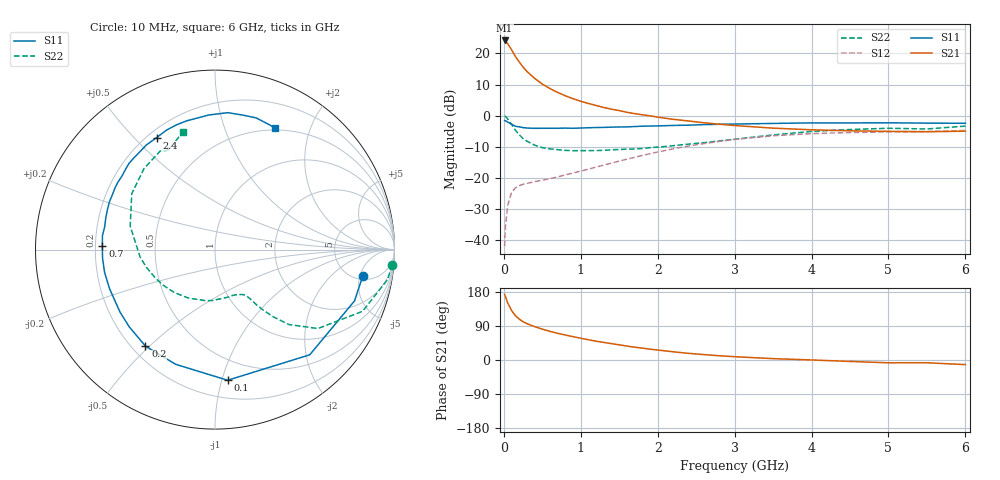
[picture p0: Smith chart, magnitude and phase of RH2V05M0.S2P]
! SIEMENS Small Signal Semiconductors
! BFR106
! Si NPN RF Bipolar Junction Transistor in SOT23
! VCE = 2 V  IC = 5 mA
! Common Emitter S-Parameters:  August  1996
# GHz  S  MA  R  50
!  f  S11  S21  S12  S22
! GHz  MAG  ANG  MAG  ANG  MAG  ANG  MAG  ANG
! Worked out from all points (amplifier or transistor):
!   36 points, 10 MHz to 6 GHz, reference 50 ohm
!   highest |S21| = 24.2 dB at 10 MHz (marker M1)
!   |S21| within 3 dB of that: start of sweep to 100.4 MHz
!   unconditionally stable (mu >= 1): 608.3 MHz to 2.204 GHz; 4.196 GHz to end of sweep
!   at 250 MHz: K = 0.51, MSG = 18.8 dB, |S12| = -22.1 dB
!   at 1.4 GHz: K = 1.17, MAG = 6.2 dB, |S12| = -15.2 dB
!   at 6 GHz: K = 1.03, MAG = -1.1 dB, |S12| = -4.7 dB
!   S11 on the Smith chart (normalised r, x): 10 MHz: 5.59, -5.56; 100 MHz: 0.33, -1.04; 200 MHz: 0.25, -0.49; 700 MHz: 0.23, +0.02; 2.4 GHz: 0.24, +0.58; 6 GHz: 0.48, +1.50
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0.01  0.8362 -10.3  16.19 173.1  0.008 87.6  0.9906 -4.9
0.02  0.8282 -20.2  15.84 167.8  0.016 80.0  0.9764 -9.8
0.05  0.7888 -48.0  14.34 150.7  0.0362 66.2  0.8911 -22.7
0.1  0.7313 -84.5  11.48 130.8  0.0583 51.0  0.7225 -37.5
0.15  0.6756 -109.0  8.952 116.8  0.0692 42.0  0.5864 -45.4
0.2  0.6627 -125.8  7.302 108.0  0.075 37.8  0.4952 -49.1
0.25  0.643 -138.0  6.043 100.9  0.0789 35.9  0.4281 -51.5
0.3  0.6336 -146.6  5.141 96.0  0.0817 35.5  0.3898 -52.9
0.4  0.6266 -159.7  3.982 88.1  0.0872 36.3  0.3362 -54.5
0.5  0.6282 -168.4  3.223 81.4  0.0918 38.5  0.3065 -56.2
0.6  0.6283 -175.9  2.726 75.6  0.0974 41.0  0.2925 -58.7
0.7  0.6281 178.1  2.366 70.4  0.104 44.0  0.2846 -61.9
0.9  0.6277 168.6  1.872 61.5  0.1199 48.9  0.2738 -68.6
1.1  0.6399 159.3  1.571 53.4  0.1384 52.8  0.2746 -77.7
1.3  0.6485 151.8  1.354 46.3  0.161 55.3  0.2773 -86.8
1.6  0.6609 141.6  1.133 36.7  0.2002 56.7  0.29 -101.9
2.2  0.697 123.3  0.875 21.7  0.2929 52.7  0.3295 -133.4
2.4  0.704 117.5  0.822 17.6  0.3254 50.0  0.3492 -145.0
3.5  0.7508 92.6  0.631 3.6  0.4758 30.3  0.4903 164.5
4.5  0.7653 78.2  0.572 -3.8  0.5356 12.2  0.5999 131.3
5.5  0.7595 67.2  0.552 -7.3  0.5569 1.6  0.6119 115.1
6  0.7556 63.7  0.564 -12.2  0.5805 -5.8  0.6803 105.2
